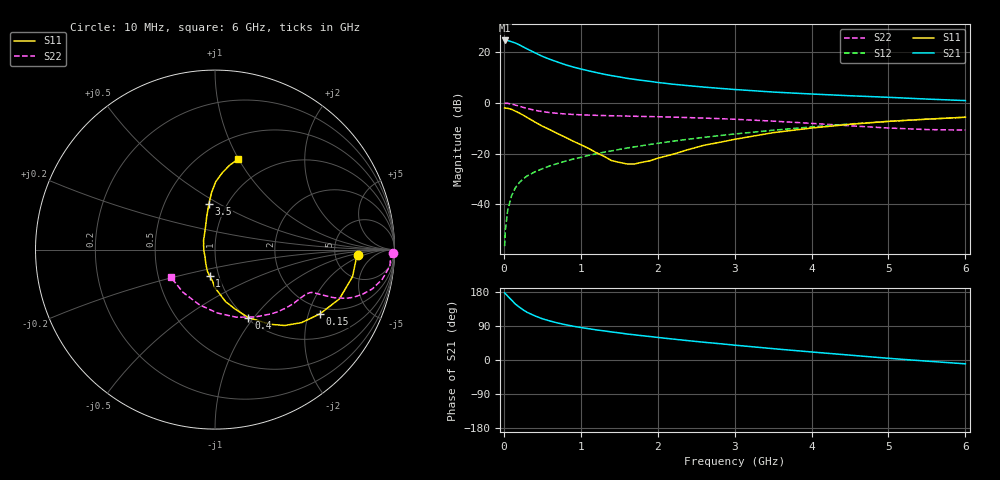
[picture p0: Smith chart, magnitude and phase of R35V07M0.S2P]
! SIEMENS Small Signal Semiconductors
! BFR181
! Si NPN RF Bipolar Junction Transistor in SOT23
! VCE = 5 V  IC = 7 mA
! Common Emitter S-Parameters:  May  1996
# GHz  S  MA  R  50
!  f  S11  S21  S12  S22
! GHz  MAG  ANG  MAG  ANG  MAG  ANG  MAG  ANG
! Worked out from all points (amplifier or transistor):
!   36 points, 10 MHz to 6 GHz, reference 50 ohm
!   highest |S21| = 24.6 dB at 10 MHz (marker M1)
!   |S21| within 3 dB of that: start of sweep to 281.6 MHz
!   unconditionally stable (mu >= 1): 966.4 MHz to 2.863 GHz
!   at 250 MHz: K = 0.49, MSG = 26.0 dB, |S12| = -30.0 dB
!   at 1.4 GHz: K = 1.05, MAG = 13.5 dB, |S12| = -18.9 dB
!   at 6 GHz: K = 0.86, MSG = 3.3 dB, |S12| = -5.7 dB
!   S11 on the Smith chart (normalised r, x): 10 MHz: 8.49, -1.47; 150 MHz: 1.76, -2.38; 400 MHz: 1.02, -0.94; 1 GHz: 0.90, -0.27; 3.5 GHz: 0.82, +0.45; 6 GHz: 0.72, +1.00
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0.01  0.7949 -2.3  16.96 177.3  0.0015 102.5  0.9898 -1.0
0.02  0.7876 -4.2  16.93 175.0  0.0031 84.0  0.9796 -2.1
0.05  0.781 -11.1  16.89 168.6  0.0076 85.2  0.9786 -5.3
0.1  0.7457 -21.6  16.04 158.3  0.0148 78.9  0.9472 -10.0
0.15  0.6855 -31.5  15.11 147.6  0.0212 73.8  0.904 -14.0
0.2  0.6312 -40.1  13.94 139.6  0.0267 72.2  0.8592 -16.8
0.25  0.5745 -47.4  12.7 132.5  0.0316 69.2  0.8162 -19.0
0.3  0.5175 -53.5  11.62 126.1  0.0361 67.8  0.7789 -20.4
0.4  0.4221 -63.9  9.778 116.8  0.0434 66.2  0.7157 -22.0
0.5  0.3479 -71.5  8.257 108.9  0.0503 66.2  0.6718 -22.6
0.6  0.2951 -78.6  7.196 102.9  0.0573 65.7  0.6426 -23.0
0.7  0.2475 -84.0  6.359 97.7  0.064 66.5  0.6208 -23.3
0.8  0.2099 -90.6  5.646 93.2  0.0709 66.6  0.6041 -23.5
1  0.1501 -101.6  4.651 85.8  0.0842 67.2  0.5819 -24.3
1.1  0.1272 -109.6  4.286 82.7  0.092 67.4  0.5742 -25.0
1.3  0.0888 -125.8  3.673 76.9  0.1065 67.0  0.5626 -26.4
1.6  0.0626 -168.3  3.05 68.7  0.1288 66.4  0.5486 -29.2
2.2  0.0973 127.8  2.33 55.2  0.1759 64.0  0.5229 -36.4
3.5  0.2585 97.5  1.633 29.9  0.2886 54.2  0.4365 -59.4
4.5  0.378 89.4  1.38 12.8  0.3844 43.7  0.3531 -88.1
5.5  0.4769 80.2  1.187 -3.0  0.478 31.2  0.2975 -126.6
6  0.5213 75.5  1.109 -10.1  0.5205 24.3  0.2907 -148.3
